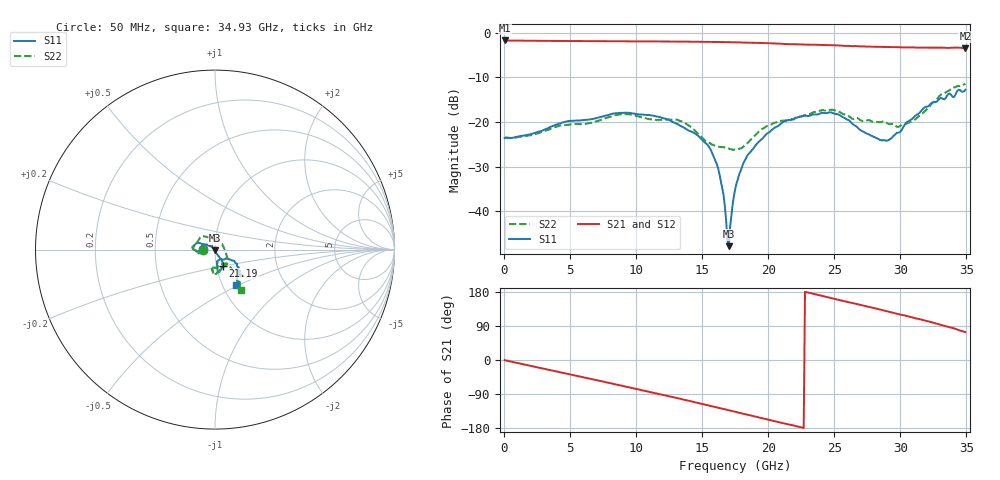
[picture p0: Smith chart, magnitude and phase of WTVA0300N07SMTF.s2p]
! 50 ohm 2-Port S-parameters measured by Modelithics Inc support@modelithics.com  Tampa, FL USA 813-866-6335 (February 2024)
! Smiths Interconnect,  3dB P/N: WTVA0300N07SMTF, Temperature: 125 C
! Board: 10 mil Rogers 4350B, Mounting Pad Dimensions: Length: 15 mils, Width: 25 mils, Gap: 40 mils.
# Hz S RI R 50
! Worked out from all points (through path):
!   352 points, 50 MHz to 34.93 GHz, reference 50 ohm
!   highest |S21| = -1.70 dB at 100 MHz (marker M1); lowest = -3.4 dB at 34.93 GHz (marker M2)
!   group delay of S21, straight-line fit = 22.5 ps
!   lowest |S11| = -47.8 dB at 17.02 GHz (marker M3), VSWR 1.01, Z = 49.8 - j0.334 ohm
!   |S11| at or under -10 dB: start of sweep to end of sweep
!   |S22| runs from -26.2 to -11.4 dB; largest |S21 - S12| = 0.0097
!   S11 on the Smith chart (normalised r, x): 50 MHz: 0.88, +0.00; 21.19 GHz: 1.07, -0.20; 34.93 GHz: 1.15, -0.49
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5e7  -0.0662 0.00124  0.8226 -0.00538  0.8216 -0.00519  -0.0658 -0.000145
1e8  -0.067 0.000402  0.8226 -0.0117  0.8218 -0.0118  -0.0668 -0.000203
5.8715e9  -0.1046 -0.00618  0.5771 -0.5679  0.5762 -0.5674  -0.0934 -0.017
8.956e9  -0.1264 0.0127  0.3017 -0.7456  0.3001 -0.7448  -0.1228 0.00539
1.1742e10  -0.1106 0.0288  0.00622 -0.8012  0.00419 -0.8  -0.0915 0.054
1.3533e10  -0.0806 0.0357  -0.1921 -0.7766  -0.194 -0.7751  -0.0672 0.0753
1.56225e10  -0.0419 0.0273  -0.4098 -0.6805  -0.4111 -0.6779  0.00294 0.0577
1.612e10  -0.0273 0.0197  -0.456 -0.6481  -0.4568 -0.6461  0.0185 0.0506
1.6518e10  -0.0142 0.0118  -0.4908 -0.6189  -0.4919 -0.6166  0.0294 0.0436
1.6717e10  -0.00954 0.00652  -0.5078 -0.6035  -0.5086 -0.6014  0.0339 0.0395
1.6916e10  -0.0047 -0.000416  -0.5242 -0.5876  -0.5243 -0.5856  0.0374 0.0348
1.70155e10  -0.0023 -0.00335  -0.532 -0.5797  -0.5322 -0.5779  0.039 0.0325
1.72145e10  0.002 -0.00881  -0.5475 -0.5645  -0.5486 -0.5616  0.0417 0.0267
1.7513e10  0.00545 -0.0172  -0.5714 -0.5381  -0.5713 -0.5363  0.0448 0.0202
1.84085e10  0.0205 -0.0367  -0.63 -0.4551  -0.6299 -0.4535  0.0573 -0.00945
2.11945e10  0.044 -0.0916  -0.7347 -0.1653  -0.7337 -0.164  0.0556 -0.0882
2.33835e10  0.0273 -0.1186  -0.7338 0.0631  -0.7328 0.0636  0.012 -0.1278
2.5274e10  0.0152 -0.1211  -0.6762 0.2584  -0.6748 0.2585  -0.00945 -0.1323
2.91545e10  0.0332 -0.0537  -0.421 0.5527  -0.4143 0.556  0.0156 -0.0936
2.9851e10  0.055 -0.0527  -0.3574 0.5919  -0.3528 0.5929  0.0351 -0.0813
3.1841e10  0.1229 -0.0788  -0.1688 0.6624  -0.1645 0.6619  0.0867 -0.099
3.49255e10  0.1149 -0.1998  0.1895 0.6454  0.1906 0.6434  0.1431 -0.2268
